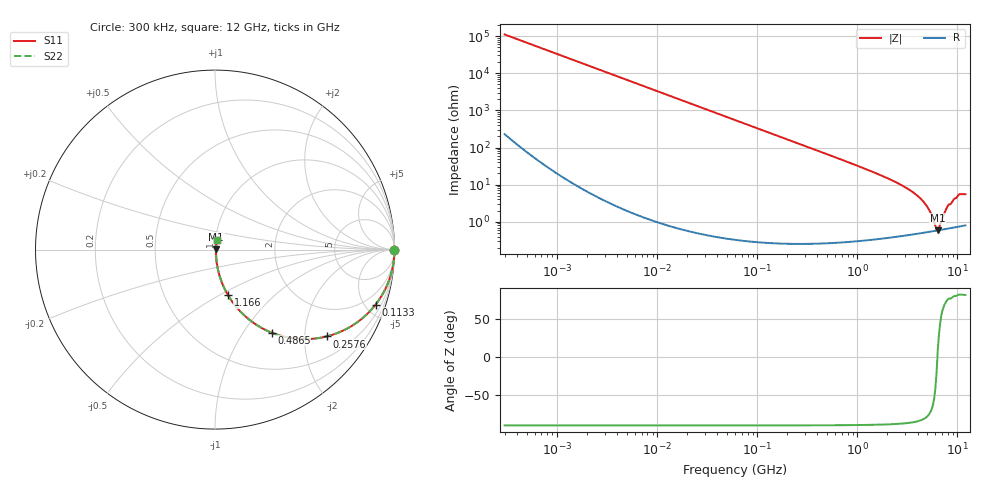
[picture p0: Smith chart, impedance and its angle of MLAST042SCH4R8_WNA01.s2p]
! MLAST042SCH4R8_WNA01  S-PARAMETER MODEL  ( General Type )
! Model Generated by TAIYO YUDEN Corporation (http://www.ty-top.com)
! Version 1.0
! TAIYO YUDEN Control No. 150820
! Copyright(c) 2015 TAIYO YUDEN CO.,LTD. All Rights Reserved.
! Product Description (link to TY-COMPAS)
! https://ds.yuden.co.jp/TYCOMPAS/or/detail?pn=MLAST042SCH4R8BWNA01&u=M
! Products Name : Multilayer Ceramic Capacitors
! Characteristics :
!  Capacitance : 4.8 pF , Rated Voltage : 25V , TCC : CH / C0H
!  Case Size : 0.4 x 0.2 / 0.016 x 0.008 [mm/inch] , Thickness : 0.2 / 0.008 [mm/inch]
!  (Conditions: Temperature = 25 degC , DC Bias Current/Voltage = 0A / 0V)
! External Node Assignments :
!  1  o---| |---o  2
! GND o---------o GND
! Frequency Range : 0.3MHz  -  12000MHz  [ 401 STEP ]
# MHz S RI R 50
! Freq[MHz].  S11 Real  S11 Imag  S21 Real  S21 Imag  S12 Real  S12 Imag  S22 Real  S22 Imag
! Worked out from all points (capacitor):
!   401 points, 300 kHz to 12 GHz, reference 50 ohm
!   read as one part in series: C = 4.8 pF near 316.3 kHz
!   lowest |Z| = 593 mohm at 6.354 GHz (marker M1)
!   series resonance near 6.305 GHz, so ESL is about 130 pH
!   S11 on the Smith chart (normalised r, x): 300 kHz: open; 113.3 MHz: 1.01, -5.85; 257.6 MHz: 1.01, -2.57; 486.5 MHz: 1.01, -1.35; 1.166 GHz: 1.01, -0.55; 12 GHz: 1.02, +0.11
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0.3  1 -0.000906  2.69e-06 0.000906  2.69e-06 0.000906  1 -0.000906
1.769972  1 -0.00534  3.08e-05 0.00534  3.08e-05 0.00534  1 -0.00534
10.44266  0.999 -0.0315  0.001 0.0315  0.001 0.0315  0.999 -0.0315
60  0.9681 -0.1753  0.0319 0.1753  0.0319 0.1753  0.9681 -0.1753
113.3117  0.895 -0.3061  0.105 0.3061  0.105 0.3061  0.895 -0.3061
168.5979  0.7937 -0.404  0.2063 0.404  0.2063 0.404  0.7937 -0.404
257.5933  0.6222 -0.4839  0.3778 0.4839  0.3778 0.4839  0.6222 -0.4839
353.9943  0.4654 -0.4974  0.5346 0.4974  0.5346 0.4974  0.4654 -0.4974
486.4723  0.3149 -0.4625  0.6851 0.4625  0.6851 0.4625  0.3149 -0.4625
743.2595  0.1635 -0.3666  0.8365 0.3666  0.8365 0.3666  0.1635 -0.3666
1166.079  0.0725 -0.2537  0.9275 0.2537  0.9275 0.2537  0.0725 -0.2537
2088.533  0.0231 -0.1375  0.9769 0.1375  0.9769 0.1375  0.0231 -0.1375
3190.978  0.0102 -0.0762  0.9898 0.0762  0.9898 0.0762  0.0102 -0.0762
4270.516  0.00663 -0.0416  0.9934 0.0416  0.9934 0.0416  0.00663 -0.0416
5140.631  0.00576 -0.0215  0.9942 0.0215  0.9942 0.0215  0.00576 -0.0215
6026.253  0.00571 -0.00481  0.9943 0.00481  0.9943 0.00481  0.00571 -0.00481
6354.153  0.00583 0.000877  0.9942 -0.000877  0.9942 -0.000877  0.00583 0.000877
6699.894  0.00601 0.00557  0.994 -0.00557  0.994 -0.00557  0.00601 0.00557
7648.807  0.00674 0.0195  0.9933 -0.0195  0.9933 -0.0195  0.00674 0.0195
8281.503  0.00743 0.0286  0.9926 -0.0286  0.9926 -0.0286  0.00743 0.0286
10511.28  0.0104 0.054  0.9896 -0.054  0.9896 -0.054  0.0104 0.054
12000  0.0109 0.0538  0.9891 -0.0538  0.9891 -0.0538  0.0109 0.0538
